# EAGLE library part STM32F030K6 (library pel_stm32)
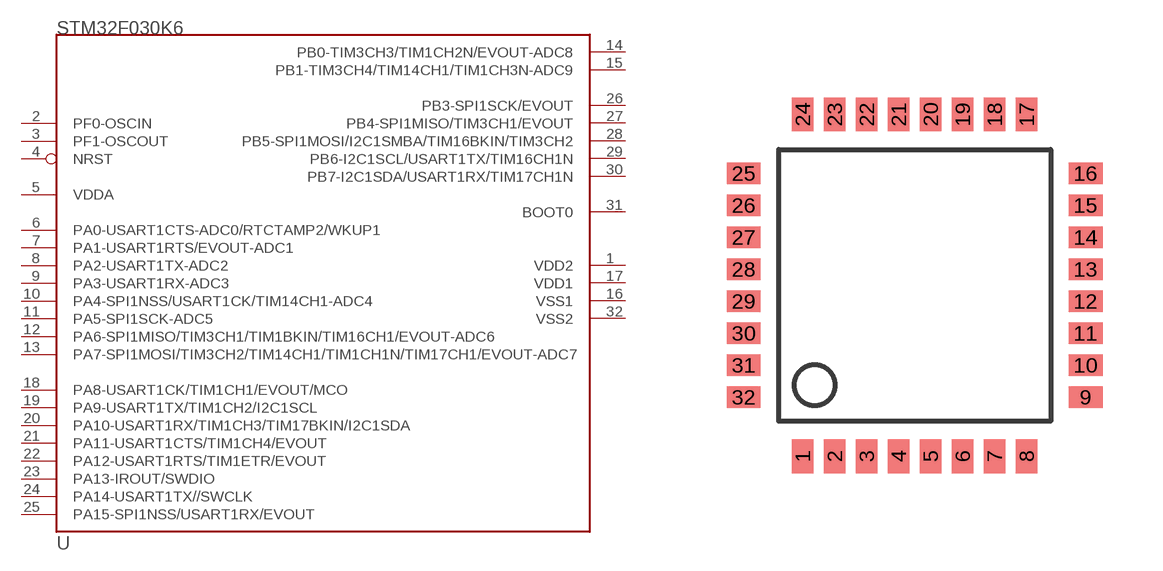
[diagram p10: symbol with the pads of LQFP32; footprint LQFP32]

Designator prefix -

## STM32F030K6  [LQFP32]
1  VDD2
2  PF0-OSCIN
3  PF1-OSCOUT
4  NRST
5  VDDA
6  PA0-USART1CTS-ADC0/RTCTAMP2/WKUP1
7  PA1-USART1RTS/EVOUT-ADC1
8  PA2-USART1TX-ADC2
9  PA3-USART1RX-ADC3
10  PA4-SPI1NSS/USART1CK/TIM14CH1-ADC4
11  PA5-SPI1SCK-ADC5
12  PA6-SPI1MISO/TIM3CH1/TIM1BKIN/TIM16CH1/EVOUT-ADC6
13  PA7-SPI1MOSI/TIM3CH2/TIM14CH1/TIM1CH1N/TIM17CH1/EVOUT-ADC7
14  PB0-TIM3CH3/TIM1CH2N/EVOUT-ADC8
15  PB1-TIM3CH4/TIM14CH1/TIM1CH3N-ADC9
16  VSS1
17  VDD1
18  PA8-USART1CK/TIM1CH1/EVOUT/MCO
19  PA9-USART1TX/TIM1CH2/I2C1SCL
20  PA10-USART1RX/TIM1CH3/TIM17BKIN/I2C1SDA
21  PA11-USART1CTS/TIM1CH4/EVOUT
22  PA12-USART1RTS/TIM1ETR/EVOUT
23  PA13-IROUT/SWDIO
24  PA14-USART1TX//SWCLK
25  PA15-SPI1NSS/USART1RX/EVOUT
26  PB3-SPI1SCK/EVOUT
27  PB4-SPI1MISO/TIM3CH1/EVOUT
28  PB5-SPI1MOSI/I2C1SMBA/TIM16BKIN/TIM3CH2
29  PB6-I2C1SCL/USART1TX/TIM16CH1N
30  PB7-I2C1SDA/USART1RX/TIM17CH1N
31  BOOT0  in
32  VSS2

## Footprint LQFP32 (pad centres in mm)
smd 0.54 x 0.85: 1 -2.8,-4.275; 2 -2,-4.275; 3 -1.2,-4.275; 4 -0.4,-4.275; 5 0.4,-4.275; 6 1.2,-4.275; 7 2,-4.275; 8 2.8,-4.275; 17 2.8,4.275; 18 2,4.275; 19 1.2,4.275; 20 0.4,4.275; 21 -0.4,4.275; 22 -1.2,4.275; 23 -2,4.275; 24 -2.8,4.275
smd 0.85 x 0.54: 9 4.275,-2.8; 10 4.275,-2; 11 4.275,-1.2; 12 4.275,-0.4; 13 4.275,0.4; 14 4.275,1.2; 15 4.275,2; 16 4.275,2.8; 25 -4.275,2.8; 26 -4.275,2; 27 -4.275,1.2; 28 -4.275,0.4; 29 -4.275,-0.4; 30 -4.275,-1.2; 31 -4.275,-2; 32 -4.275,-2.8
